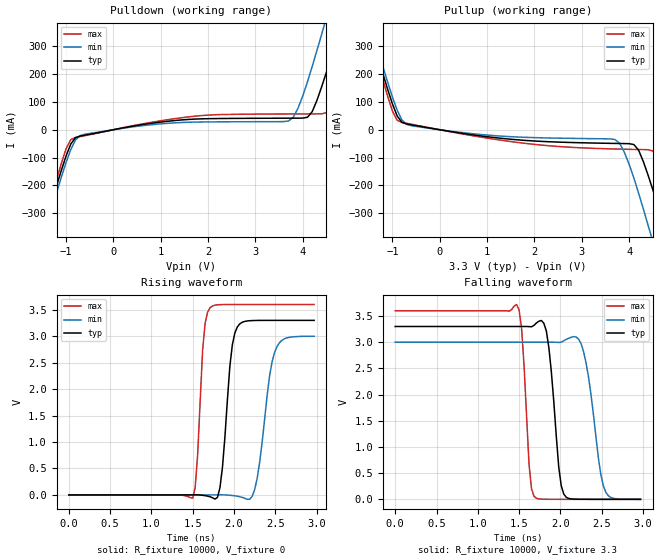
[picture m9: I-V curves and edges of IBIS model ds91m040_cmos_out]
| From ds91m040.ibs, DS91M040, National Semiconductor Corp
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|   Model  ds91m040_cmos_out
[Model]   ds91m040_cmos_out
Model_type Output
Polarity Non-Inverting
Vref=1.65
Vmeas=1.65
C_comp   4.274p  3.974p  4.595p
[Temperature Range]   25   85   -40
[Voltage Range]   3.3   3.0   3.6
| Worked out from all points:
|   slope of the pulldown table from 0 to 0.495 V, typ, clamps not added: 32.4 ohm
|   slope of the pullup table from 0 to 0.495 V, typ, clamps not added: 36.9 ohm
|   rising waveform, R_fixture 10000, V_fixture 0: 20-80 % time 97.9ps typ, 139ps min, 70.6ps max; typ from 0 V to 3.3 V
|   falling waveform, R_fixture 10000, V_fixture 3.3: 20-80 % time 101ps typ, 144ps min, 72.2ps max; typ from 3.3 V to 0 V
[Pullup]
|Vtable   (typ)   I(min)   I(max)
-3.3V     1.541A     1.502A     1.369A
-1.5V     382.7mA    402.6mA    364mA
-900mV    49.7mA     70.73mA    33.97mA
-700mV    20.75mA    19.31mA    23.13mA
1.971fV   24.11pA    43.41pA    22.1pA
3.7V      -49.29mA   -35.24mA   -69.29mA
3.9V      -49.82mA   -81.18mA   -70.13mA
4.2V      -73.64mA   -228.4mA   -71.2mA
4.5V      -215.8mA   -402.9mA   -76.38mA
4.8V      -384.8mA   -583.2mA   -212.3mA
5.1V      -572.7mA   -765.8mA   -388.4mA
6.5V      -1.478A    -1.506A    -1.301A
[Pulldown]
|V(pulldown)   I(typ)   I(min)   I(max)
-3.3V     -1.543A    -1.506A    -1.573A
-1.5V     -382.5mA   -402.4mA   -365.2mA
-1V       -95.28mA   -118.6mA   -69.05mA
-700mV    -22.65mA   -20.88mA   -24.75mA
1.7V      38.18mA    27.43mA    48.33mA
3.7V      41.6mA     31.49mA    56.75mA
3.9V      41.71mA    77.24mA    56.89mA
4.2V      64.95mA    227.9mA    57.09mA
4.5V      206.7mA    402.8mA    61.54mA
4.8V      383.2mA    583.1mA    196.8mA
5.1V      572.5mA    765.4mA    372.5mA
6.5V      1.476A     1.626A     1.301A
[Rising Waveform]
R_fixture= 10000
V_fixture= 0
V_fixture_min= 0
V_fixture_max= 0
0s        637.9pV    1.177nV    552.3pV
1.5ns     492.2uV    3.771uV    -62.28mV
1.56ns    1.5mV      -13.18uV   764.7mV
1.65ns    -14.69mV   -56.21uV   3.243V
1.8ns     -47.23mV   797.3uV    3.594V
1.98ns    2.838V     -11.78mV   3.6V
2.19ns    3.293V     -80.95mV   3.6V
2.28ns    3.299V     311.2mV    3.6V
2.49ns    3.3V       2.689V     3.6V
2.97ns    3.3V       2.999V     3.6V
|3.0E-9   3.3000   2.9997   3.6000
[Falling Waveform]
R_fixture=10000
V_fixture=3.3
V_fixture_min=3.0
V_fixture_max=3.6
0s        3.3V       3V         3.6V
1.47ns    3.3V       3V         3.72V
1.53ns    3.3V       3V         3.264V
1.65ns    3.294V     3V         204.1mV
1.77ns    3.414V     3V         3.659mV
1.86ns    2.897V     3V         827.2uV
2.01ns    259.8mV    3.001V     83.85uV
2.19ns    2.833mV    3.099V     4.8uV
2.55ns    66.12uV    133.8mV    15.77nV
2.97ns    926.1nV    528uV      570.8pV
|3.0E-9   6.8268E-7   4.3004E-4   5.6369E-10
[Ramp]
|   typ   min   max
dV/dt_r   1.98V/0.095ns   1.8V/0.137ns   2.16V/0.068ns
dV/dt_f   1.98V/0.099ns   1.8V/0.142ns   2.16V/0.070ns
R_load=50
|[End]  ds91m040_cmos_out
